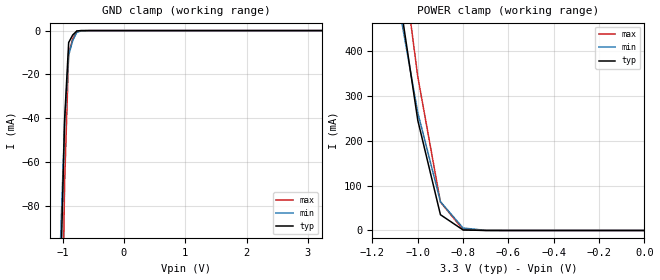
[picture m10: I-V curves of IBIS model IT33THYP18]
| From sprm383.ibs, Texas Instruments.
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|   Model Cell IT33THYP18
[Model]   IT33THYP18
Model_type   Input
Polarity   Non-Inverting
Vinl =  0.8V
Vinh =  2V
C_comp   0.4844409p   0.438389p   0.5468824p
[Model Spec]
Vinl   0.8V   0.8V   0.8V
Vinh   2V   2V   2V
[Temperature Range]   25   105   0
[Voltage Range]   3.3   3.14   3.47
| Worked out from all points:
|   GND clamp passes 1 mA (typ) near -0.80 V on its own axis
|   POWER clamp passes 1 mA (typ) near -0.79 V on its own axis
[POWER_clamp]
|   voltage   I(typ)   I(min)   I(max)
-3.3V     9.936A     8.589A     10.91A
-1.067V   472mA      454mA      602.8mA
-1.033V   359.1mA    358.5mA    473.2mA
-1V       246.2mA    263mA      343.5mA
-900mV    35.2mA     64.25mA    63.47mA
-800mV    1.114mA    5.423mA    1.777mA
-700mV    25.93uA    322.4uA    29.63uA
-11.55fV  94.85nA    66.15nA    457.2nA
[GND_clamp]
|   voltage   I(typ)   I(min)   I(max)
-3.3V     -13.46A    -11.58A    -14.63A
-1.033V   -115.4mA   -96.26mA   -194mA
-966.7mV  -40.87mA   -42.82mA   -70.17mA
-900mV    -5.431mA   -11.17mA   -10.32mA
-833.3mV  -1.981mA   -4.449mA   -3.622mA
-766.7mV  -175.5uA   -788.7uA   -186uA
-700mV    -14.39uA   -190.2uA   -14.64uA
-500mV    -1.186uA   -1.487uA   -2.672uA
3.233V    93.61nA    67.2nA     435nA
